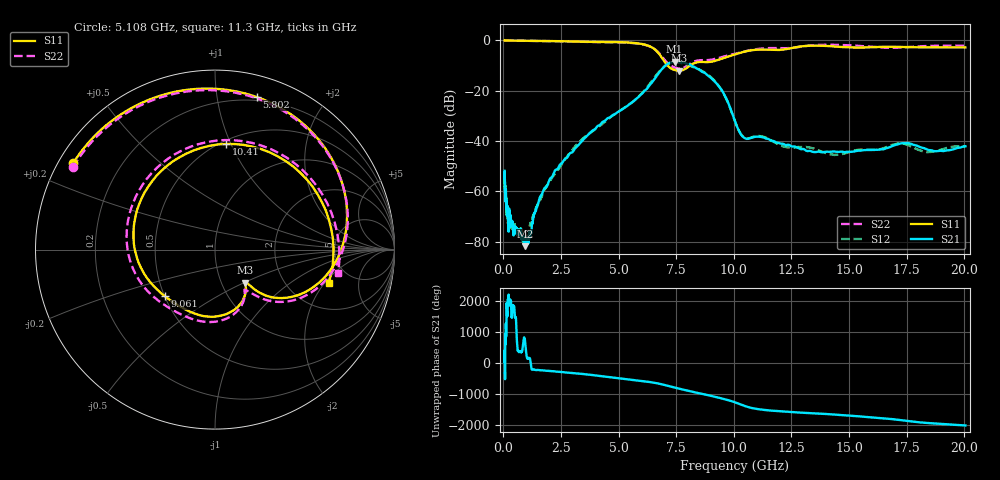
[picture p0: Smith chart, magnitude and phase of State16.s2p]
# Hz S DB R 50
!freq MagS11 AngS11 MagS21 AngS21 MagS12 AngS12 MagS22 AngS22
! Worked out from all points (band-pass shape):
!   1601 points, 50 MHz to 20.05 GHz, reference 50 ohm
!   highest |S21| = -8.46 dB at 7.43 GHz (marker M1); lowest = -81.7 dB at 943 MHz (marker M2)
!   |S21| within 3 dB of the highest: 6.868 GHz to 8.481 GHz (1.613 GHz wide, 21 % of centre)
!   lowest |S11| = -12.0 dB at 7.627 GHz (marker M3), VSWR 1.67, Z = 64.5 - j25.4 ohm
!   |S11| at or under -10 dB: 7.129 GHz to 8.093 GHz (963.5 MHz wide, 12.7 % of centre)
!   |S22| runs from -11.2 to 0.0 dB; largest |S21 - S12| = 0.02
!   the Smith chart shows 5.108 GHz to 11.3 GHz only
!   S11 on the Smith chart (normalised r, x): 5.108 GHz: 0.04, +0.28; 5.802 GHz: 0.17, +1.30; 9.061 GHz: 0.50, -0.31; 10.41 GHz: 0.53, +0.96; 11.3 GHz: 3.34, -2.21
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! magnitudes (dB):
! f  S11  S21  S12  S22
! 50 MHz  0.0  -51.8  -57.3  0.0
! 82.91 MHz  0.0  -63.4  -61.0  0.0
! 103.8 MHz  0.0  -59.3  -62.0  0.0
! 135.9 MHz  0.0  -64.5  -66.6  0.0
! 188.3 MHz  0.0  -66.9  -71.5  0.0
! 222.9 MHz  0.0  -76.0  -73.8  0.0
! 248.5 MHz  0.0  -68.2  -72.9  0.0
! 286.5 MHz  0.0  -73.4  -73.4  0.0
! 369.6 MHz  0.0  -72.7  -73.5  0.0
! 943 MHz  -0.1  -81.7  -79.1  -0.1
! 1.005 GHz  -0.1  -79.6  -78.2  -0.1
! 2.722 GHz  -0.3  -46.8  -46.7  -0.4
! 5.108 GHz  -0.7  -27.7  -27.6  -0.8
! 5.802 GHz  -1.1  -22.9  -22.9  -1.2
! 7.402 GHz  -11.7  -8.5  -8.8  -10.6
! 7.43 GHz  -11.7  -8.5  -8.8  -10.7
! 7.627 GHz  -12.0  -8.5  -8.8  -11.2
! 9.061 GHz  -8.4  -15.3  -15.0  -7.6
! 10.41 GHz  -4.6  -38.4  -38.3  -4.4
! 11.3 GHz  -3.6  -38.6  -38.3  -3.1
! 14.37 GHz  -2.4  -44.1  -45.5  -1.7
! 20.05 GHz  -2.8  -42.0  -42.1  -2.1
